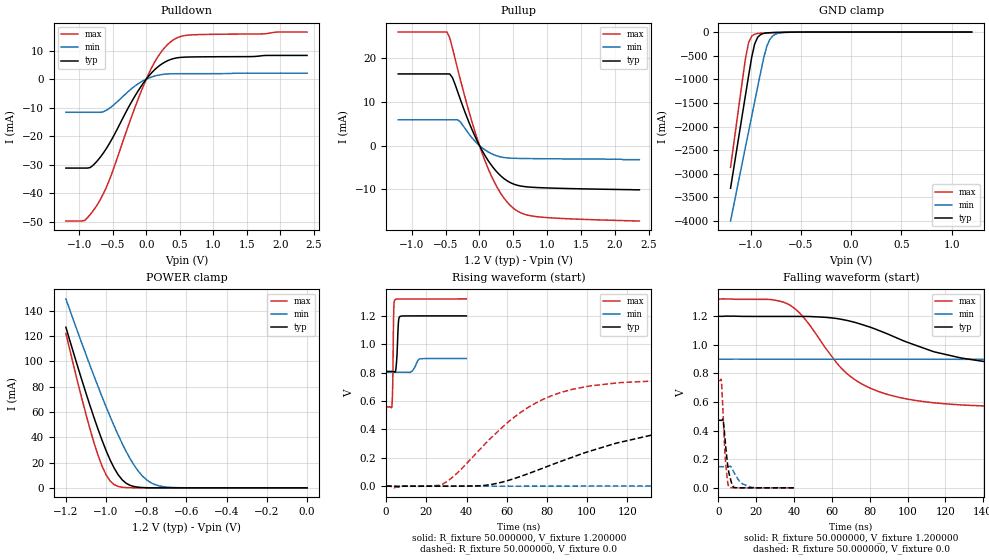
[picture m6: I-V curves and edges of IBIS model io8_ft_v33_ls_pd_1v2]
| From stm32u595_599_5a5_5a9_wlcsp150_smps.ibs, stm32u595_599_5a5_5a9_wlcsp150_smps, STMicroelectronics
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|   Model io8_ft_v33_ls_pd_1v2
[Model]  io8_ft_v33_ls_pd_1v2
Model_type I/O
Polarity   Non-Inverting
Enable   Active-Low
Vinl =   0.360000V
Vinh =   0.840000V
Vmeas =  0.600000V
Cref =   50.000000pF
Rref =   100.000000M
Vref =   0.0V
C_comp   2.887200pF   2.816900pF   2.935200pF
[Temperature Range]   25.000000   0.140000k   -40.000000
[Pullup Reference]   1.200000V   0.900000V   1.320000V
[Pulldown Reference]   0.0V   0.0V   0.0V
[POWER Clamp Reference]   1.200000V   0.900000V   1.320000V
[GND Clamp Reference]   0.0V   0.0V   0.0V
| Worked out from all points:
|   slope of the pulldown table from 0 to 0.18 V, typ, clamps not added: 40.7 ohm
|   slope of the pullup table from 0 to 0.18 V, typ, clamps not added: 39.5 ohm
|   GND clamp passes 1 mA (typ) near -0.51 V on its own axis
|   POWER clamp passes 1 mA (typ) near -0.86 V on its own axis
|   rising waveform, R_fixture 50.000000, V_fixture 1.200000: 20-80 % time 751ps typ, 2.06ns min, 413ps max; typ from 0.808 V to 1.2 V
|   rising waveform, R_fixture 50.000000, V_fixture 0.0: 20-80 % time 67.6ns typ, 169ns min, 37.1ns max; typ from 0 V to 0.472 V
|   falling waveform, R_fixture 50.000000, V_fixture 1.200000: 20-80 % time 58.3ns typ, 150ns min, 31.6ns max; typ from 1.2 V to 0.808 V
|   falling waveform, R_fixture 50.000000, V_fixture 0.0: 20-80 % time 2.49ns typ, 4.76ns min, 1.84ns max; typ from 0.472 V to 0 V
[Pulldown]
|Voltage   I(typ)   I(min)   I(max)
-1.2V     -31.16mA   -11.61mA   -49.71mA
-920mV    -31.16mA   -11.61mA   -49.48mA
-840mV    -31mA      -11.61mA   -47.54mA
-720mV    -28.33mA   -11.61mA   -43.58mA
-560mV    -22.95mA   -10.37mA   -35.89mA
-200mV    -7.146mA   -2.964mA   -11.89mA
0V        0A         -100fA     -10fA
160mV     4.047mA    1.298mA    7.361mA
360mV     6.87mA     1.87mA     13mA
480mV     7.543mA    1.91mA     14.69mA
640mV     7.765mA    1.923mA    15.46mA
2.4V      8.316mA    2.102mA    16.52mA
[Pullup]
|Voltage   I(typ)   I(min)   I(max)
-1.2V     16.39mA    5.9mA      25.96mA
-480mV    16.39mA    5.9mA      25.96mA
-440mV    16.39mA    5.9mA      24.63mA
-400mV    15.57mA    5.9mA      22.35mA
-320mV    12.21mA    5.9mA      17.37mA
-120mV    3.997mA    1.962mA    5.905mA
80mV      -2.237mA   -962.6uA   -3.434mA
280mV     -6.404mA   -2.453mA   -10.06mA
520mV     -8.88mA    -2.901mA   -14.54mA
680mV     -9.389mA   -2.951mA   -15.76mA
920mV     -9.627mA   -2.991mA   -16.35mA
2.36V     -10.1mA    -3.2mA     -17.23mA
[GND_clamp]
|Voltage   I(typ)   I(min)   I(max)
-1.2V     -3.305A    -3.998A    -2.862A
-1.05V    -1.316A    -2.418A    -539.3mA
-1.02V    -921mA     -2.103A    -218.8mA
-990mV    -539.5mA   -1.788A    -87.45mA
-960mV    -252.2mA   -1.474A    -44.37mA
-930mV    -110.5mA   -1.16A     -30.33mA
-870mV    -28.04mA   -549.1mA   -21.1mA
-840mV    -18.44mA   -305.6mA   -18.29mA
-810mV    -13.92mA   -159.7mA   -15.75mA
-780mV    -11.24mA   -82.36mA   -13.39mA
-600mV    -2.986mA   -4.279mA   -3.072mA
1.2V      30.28uA    18.17uA    37.27uA
[POWER_clamp]
|Voltage   I(typ)   I(min)   I(max)
-1.2V     127mA      149.4mA    122.2mA
-1.12V    84.97mA    114mA      70.27mA
-1.06V    55.51mA    88.42mA    35.67mA
-1.02V    37.63mA    72.04mA    17.17mA
-1V       29.51mA    64.13mA    10.3mA
-960mV    15.69mA    48.99mA    2.571mA
-900mV    3.624mA    28.77mA    182.8uA
-840mV    490.7uA    13.24mA    11.35uA
-800mV    116.8uA    6.532mA    1.77uA
-740mV    13.2uA     1.723mA    109.1nA
-620mV    167.3nA    79.35uA    0A
0V        0A         17.84nA    0A
[Ramp]
| variable   typ   min   max
dV/dt_r  0.28339/67.48888n   88.78188m/0.16835u  0.45041/37.05944n
dV/dt_f  0.23487/58.20219n   58.03200m/0.14998u  0.45673/31.57339n
R_load = 50.000000
[Rising Waveform]
R_fixture= 50.000000
V_fixture= 1.200000
V_fixture_min= 0.900000
V_fixture_max= 1.320000
|time   V(typ)   V(min)   V(max)
0s        808mV      802.7mV    558.2mV
2.883ns   808.1mV    802.7mV    567.5mV
3.283ns   808mV      802.7mV    729.7mV
3.764ns   806.5mV    802.7mV    1.236V
4.324ns   803.4mV    802.7mV    1.312V
5.125ns   867.2mV    802.7mV    1.317V
6.166ns   1.163V     802.7mV    1.318V
6.807ns   1.194V     802.7mV    1.318V
16.98ns   1.199V     896.8mV    1.319V
39.88ns   1.199V     899.4mV    1.319V
[Rising Waveform]
R_fixture= 50.000000
V_fixture= 0.0
V_fixture_min= 0.0
V_fixture_max= 0.0
|time   V(typ)   V(min)   V(max)
0s        2.199nV    207.3nV    1.402nV
28.03ns   -71.37uV   -26.39uV   13.99mV
52.05ns   10.76mV    -20.35uV   338mV
72.07ns   95.09mV    3.774uV    566.5mV
92.09ns   201mV      73.44uV    680.1mV
118.1ns   314.5mV    425.2uV    730.7mV
170.2ns   429.5mV    7.387mV    749.5mV
254.3ns   468mV      55.17mV    750.8mV
452.5ns   472.3mV    134.7mV    750.7mV
997ns     472.4mV    148.1mV    750.8mV
[Falling Waveform]
R_fixture= 50.000000
V_fixture= 1.200000
V_fixture_min= 0.900000
V_fixture_max= 1.320000
|time   V(typ)   V(min)   V(max)
0s        1.199V     899.4mV    1.319V
36.04ns   1.198V     899.1mV    1.289V
44.04ns   1.198V     899.1mV    1.207V
64.06ns   1.181V     899.1mV    849.1mV
76.08ns   1.141V     899.1mV    724.5mV
98.1ns    1.027V     899.1mV    625.3mV
130.1ns   904.3mV    898.6mV    578.5mV
256.3ns   813.6mV    859.7mV    558.3mV
444.4ns   808.1mV    811.9mV    558.2mV
997ns     808mV      802.7mV    558.2mV
[Falling Waveform]
R_fixture= 50.000000
V_fixture= 0.0
V_fixture_min= 0.0
V_fixture_max= 0.0
|time   V(typ)   V(min)   V(max)
0s        472.4mV    148.1mV    750.8mV
1.522ns   472mV      148.1mV    749.6mV
2.402ns   478.5mV    148.1mV    526.5mV
3.524ns   332.3mV    148.1mV    218mV
4.725ns   174.1mV    147.8mV    54.51mV
5.365ns   114.4mV    149.1mV    9.162mV
8.569ns   1.679mV    99.01mV    269.1uV
11.93ns   292.5uV    35.48mV    -24.67uV
17.54ns   -804.9nV   3.438mV    -34.5uV
39.88ns   2.199nV    207.3nV    1.402nV
